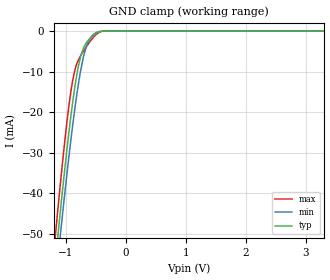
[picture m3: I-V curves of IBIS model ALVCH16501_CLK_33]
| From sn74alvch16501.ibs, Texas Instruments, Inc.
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[Model]   ALVCH16501_CLK_33
Model_type  Input
Vinl=0.8
Vinh=2.0
| variable   typ   min   max
C_comp   1.11pF   0.80pF   1.26pF
[Temperature Range]   40   100   -40
| Ambient temperature   25   85   -40
[Voltage range]   3.3   3   3.6
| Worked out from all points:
|   GND clamp passes 1 mA (typ) near -0.53 V on its own axis
[GND Clamp]
| ALVCH16501_CLK_33
|   Voltage   I(typ)   I(min)   I(max)
-3.3V     -412.4mA   -407.9mA   -421.5mA
-1.18V    -57.67mA   -63.23mA   -51.41mA
-1.155V   -53.91mA   -59.57mA   -47.5mA
-1.135V   -50.94mA   -56.66mA   -44.41mA
-1.095V   -45.07mA   -50.93mA   -38.33mA
-1.075V   -42.19mA   -48.1mA    -35.37mA
-920mV    -21.52mA   -27.44mA   -15.38mA
-860mV    -14.84mA   -20.33mA   -10.36mA
-790mV    -8.686mA   -13.06mA   -7.132mA
-655mV    -2.832mA   -3.759mA   -3.838mA
-495mV    -604.1uA   -406.3uA   -878.7uA
3.3V      919.4pA    48.35nA    20.01pA
